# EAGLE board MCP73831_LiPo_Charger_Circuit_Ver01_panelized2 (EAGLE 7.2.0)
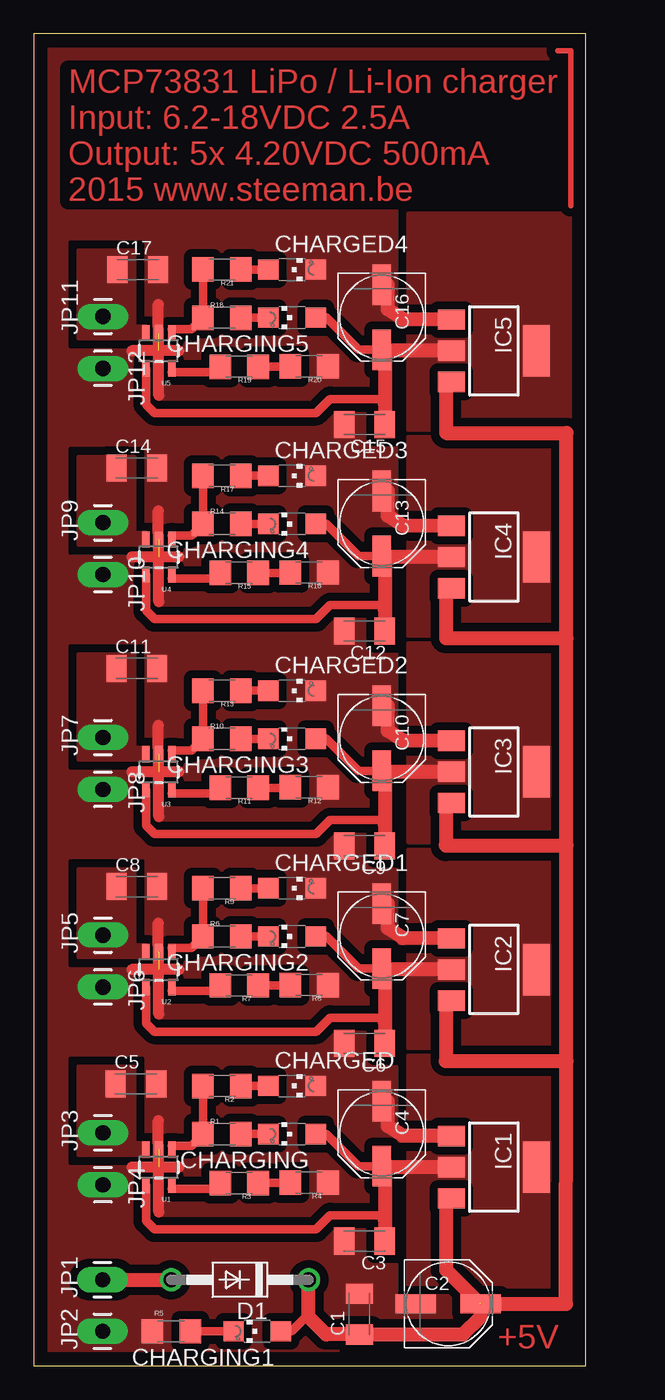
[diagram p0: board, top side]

Size 40.81 x 98.42 mm. Coordinates in mm from the lower left corner, seen from the top.
Outline: 0,0 40.81,0 40.81,98.42 0,98.42 0,0
Copper layers (1*16): Top 0.035mm / dielectric 1.5mm / Bottom 0.035mm
Design rules "default": minimum track width 10mil, minimum drill 24mil, track to track 8mil, track to pad 8mil, pad to pad 8mil, via to via 8mil, smd to smd 8mil, copper to edge 40mil, drill to drill 8mil, minimum pad ring 10mil, minimum via ring 8mil, stop-mask expansion 4mil, vias tented up to drill 0mil, thermal gap 10mil

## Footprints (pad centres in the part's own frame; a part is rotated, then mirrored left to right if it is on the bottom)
C1206K = smd 1.5 x 2: 1 -1.5,0; 2 1.5,0
PANASONIC_D = smd 3 x 1.4: + 2.4,0; - -2.4,0
CHIPLED_1206 = smd 1.5 x 1.5: A 0,-1.75; C 0,1.75
DO41-10 = drill 1.118: A 5.08,0; C -5.08,0
SOT223 = smd 1.5 x 2: 1 -2.3,-3.15; 2 0,-3.15; 3 2.3,-3.15 | smd 3.8 x 2: 4 0,3.15
1X01_LONGPAD = drill 1.118 pad 1.88 long: 1 0,0
1206 = smd 1.6 x 1.8: 1 -1.4,0; 2 1.4,0
SOT23-5 = smd 0.55 x 1.2: 1 -0.95,-1.3; 2 0,-1.3; 3 0.95,-1.3; 4 0.95,1.3; 5 -0.95,1.3

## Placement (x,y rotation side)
C1  100n  [C1206K]  24.07,3.81 90 top
C2  [PANASONIC_D]  30.64,4.57 0 top
C3  100n  [C1206K]  24.45,9.21 180 top
C4  [PANASONIC_D]  25.72,17.14 270 top
C5  10µ  [C1206K]  7.56,20.83 0 top
C6  100n  [C1206K]  24.45,23.81 180 top
C7  [PANASONIC_D]  25.72,31.75 270 top
C8  10µ  [C1206K]  7.62,35.4 0 top
C9  100n  [C1206K]  24.45,38.42 180 top
C10  [PANASONIC_D]  25.72,46.35 270 top
C11  10µ  [C1206K]  7.62,51.53 0 top
C12  100n  [C1206K]  24.45,54.29 180 top
C13  [PANASONIC_D]  25.72,62.23 270 top
C14  10µ  [C1206K]  7.62,66.33 0 top
C15  100n  [C1206K]  24.45,69.53 180 top
C16  [PANASONIC_D]  25.72,77.47 270 top
C17  10µ  [C1206K]  7.68,80.99 0 top
CHARGED  [CHIPLED_1206]  19.08,20.67 270 top
CHARGED1  [CHIPLED_1206]  19.08,35.27 270 top
CHARGED2  [CHIPLED_1206]  19.08,49.88 270 top
CHARGED3  [CHIPLED_1206]  19.08,65.75 270 top
CHARGED4  [CHIPLED_1206]  19.08,80.99 270 top
CHARGING  [CHIPLED_1206]  19.08,17.11 90 top
CHARGING1  [CHIPLED_1206]  16.51,2.54 90 top
CHARGING2  [CHIPLED_1206]  19.08,31.72 90 top
CHARGING3  [CHIPLED_1206]  19.08,46.32 90 top
CHARGING4  [CHIPLED_1206]  19.08,62.2 90 top
CHARGING5  [CHIPLED_1206]  19.08,77.44 90 top
D1  1N4004  [DO41-10]  15.24,6.35 180 top
IC1  TLV1117-50IDCYR (2342579)  [SOT223]  34,14.67 270 top
IC2  TLV1117-50IDCYR (2342579)  [SOT223]  34,29.27 270 top
IC3  TLV1117-50IDCYR (2342579)  [SOT223]  34,43.88 270 top
IC4  TLV1117-50IDCYR (2342579)  [SOT223]  34,59.75 270 top
IC5  TLV1117-50IDCYR (2342579)  [SOT223]  34,74.99 270 top
JP1  M01PTH_LONGPAD  [1X01_LONGPAD]  5.08,6.35 90 top
JP2  M01PTH_LONGPAD  [1X01_LONGPAD]  5.08,2.54 90 top
JP3  M01PTH_LONGPAD  [1X01_LONGPAD]  5.11,17.21 90 top
JP4  M01PTH_LONGPAD  [1X01_LONGPAD]  5.11,13.37 270 top
JP5  M01PTH_LONGPAD  [1X01_LONGPAD]  5.11,31.81 90 top
JP6  M01PTH_LONGPAD  [1X01_LONGPAD]  5.11,27.97 270 top
JP7  M01PTH_LONGPAD  [1X01_LONGPAD]  5.11,46.42 90 top
JP8  M01PTH_LONGPAD  [1X01_LONGPAD]  5.11,42.58 270 top
JP9  M01PTH_LONGPAD  [1X01_LONGPAD]  5.11,62.29 90 top
JP10  M01PTH_LONGPAD  [1X01_LONGPAD]  5.11,58.45 270 top
JP11  M01PTH_LONGPAD  [1X01_LONGPAD]  5.11,77.53 90 top
JP12  M01PTH_LONGPAD  [1X01_LONGPAD]  5.11,73.69 270 top
R1  1K  [1206]  13.91,17.11 0 top
R2  1K  [1206]  13.91,20.67 180 top
R3  1K  [1206]  15.18,13.49 180 top
R4  1K  [1206]  20.35,13.53 180 top
R5  1K  [1206]  10.16,2.54 0 top
R6  1K  [1206]  13.91,31.72 0 top
R7  1K  [1206]  15.18,28.1 180 top
R8  1K  [1206]  20.35,28.13 180 top
R9  1K  [1206]  13.91,35.27 180 top
R10  1K  [1206]  13.91,46.32 0 top
R11  1K  [1206]  15.18,42.7 180 top
R12  1K  [1206]  20.35,42.74 180 top
R13  1K  [1206]  13.91,49.88 180 top
R14  1K  [1206]  13.91,62.2 0 top
R15  1K  [1206]  15.18,58.58 180 top
R16  1K  [1206]  20.35,58.61 180 top
R17  1K  [1206]  13.91,65.75 180 top
R18  1K  [1206]  13.91,77.44 0 top
R19  1K  [1206]  15.18,73.82 180 top
R20  1K  [1206]  20.35,73.85 180 top
R21  1K  [1206]  13.91,80.99 180 top
U1  MCP73831  [SOT23-5]  9.24,14.67 180 top
U2  MCP73831  [SOT23-5]  9.24,29.27 180 top
U3  MCP73831  [SOT23-5]  9.24,43.88 180 top
U4  MCP73831  [SOT23-5]  9.24,59.75 180 top
U5  MCP73831  [SOT23-5]  9.24,74.99 180 top

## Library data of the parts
C1-C17 = rcl
CHARGED CHARGED1-CHARGED4 CHARGING CHARGING1-CHARGING5 = adafruit
D1 = diode
IC1-IC5 = v-reg
JP1-JP12 R1-R21 U1-U5 = SparkFun

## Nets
GND: C1.2 C2.- C3.2 C4.- C5.2 C6.2 C7.- C8.2 C9.2 C10.- C11.2 C12.2 C13.- C14.2 C15.2 C16.- C17.2 CHARGED1.C CHARGED2.C CHARGED3.C CHARGED4.C CHARGED.C IC1.1 IC2.1 IC3.1 IC4.1 IC5.1 JP2.1 JP4.1 JP6.1 JP8.1 JP10.1 JP12.1 R4.1 R5.1 R8.1 R12.1 R16.1 R20.1 U1.2 U2.2 U3.2 U4.2 U5.2
LIPO: C5.1 JP3.1 U1.3
LIPO1: C8.1 JP5.1 U2.3
LIPO2: C11.1 JP7.1 U3.3
LIPO3: C14.1 JP9.1 U4.3
LIPO5: C17.1 JP11.1 U5.3
N$1: CHARGING1.C R5.2
N$2: R3.1 R4.2
N$3: CHARGING.C R1.2
N$4: R3.2 U1.5
N$5: R1.1 R2.2 U1.1
N$6: CHARGED.A R2.1
N$7: CHARGING2.C R6.2
N$8: R7.1 R8.2
N$9: R7.2 U2.5
N$10: R6.1 R9.2 U2.1
N$11: CHARGED1.A R9.1
N$12: CHARGING3.C R10.2
N$13: R11.1 R12.2
N$14: R11.2 U3.5
N$15: R10.1 R13.2 U3.1
N$16: CHARGED2.A R13.1
N$17: CHARGING4.C R14.2
N$18: R15.1 R16.2
N$19: R15.2 U4.5
N$20: R14.1 R17.2 U4.1
N$21: CHARGED3.A R17.1
N$22: CHARGING5.C R18.2
N$23: R19.1 R20.2
N$24: R19.2 U5.5
N$25: R18.1 R21.2 U5.1
N$26: CHARGED4.A R21.1
V_IN: D1.A JP1.1
V_IN_PROT: C1.1 C2.+ CHARGING1.A D1.C IC1.3 IC4.3
V_IN_PROT1: IC2.3
V_IN_PROT2: IC3.3
V_IN_PROT4: IC5.3
VCC: C3.1 C4.+ CHARGING.A IC1.2 IC1.4 U1.4
VCC1: C6.1 C7.+ CHARGING2.A IC2.2 IC2.4 U2.4
VCC2: C9.1 C10.+ CHARGING3.A IC3.2 IC3.4 U3.4
VCC3: C12.1 C13.+ CHARGING4.A IC4.2 IC4.4 U4.4
VCC5: C15.1 C16.+ CHARGING5.A IC5.2 IC5.4 U5.4

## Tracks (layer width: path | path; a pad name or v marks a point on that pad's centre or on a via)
GND  (5 unrouted)
  Top 0.813: 9.24,11.37 9.24,14.67 9.21,18.1 | 10.73,14.67 7.24,14.67 | 9.24,25.97 9.24,29.27 9.21,32.7 | 10.73,29.27 7.24,29.27 | 9.24,40.58 9.24,43.88 9.21,47.31 | 10.73,43.88 7.24,43.88 | 9.24,56.45 9.24,59.75 9.21,63.18 | 10.73,59.75 7.24,59.75 | 9.24,71.69 9.24,74.99 9.21,78.42 | 10.73,74.99 7.24,74.99
  Top 1.016: IC1.1 27.28,17 26.16,17.72 26.16,19.55 C4.- | IC2.1 27.28,31.61 26.16,32.32 26.16,34.15 C7.- | IC3.1 27.28,46.21 26.16,46.93 26.16,48.76 C10.- | IC4.1 27.28,62.09 26.16,62.8 26.16,64.63 C13.- | IC5.1 27.28,77.33 26.16,78.04 26.16,79.87 C16.-
  pour Top (isolate 0.61, rank 2, no thermals): 0,0 0,99.06 40.64,99.06 40.64,0
LIPO
  pour Top (isolate 0.254, no thermals): 8.29,15.56 3.27,15.56 3.27,22.1 7.46,22.1 7.46,16.48 8.29,16.48
LIPO1
  pour Top (isolate 0.254, no thermals): 8.29,30.16 3.27,30.16 3.27,36.7 7.46,36.7 7.46,31.08 8.29,31.08
LIPO2
  pour Top (isolate 0.254, no thermals): 8.29,44.77 3.27,44.77 3.27,52.58 7.46,52.58 7.46,45.69 8.29,45.69
LIPO3
  pour Top (isolate 0.254, no thermals): 8.29,60.64 3.27,60.64 3.27,67.18 7.46,67.18 7.46,61.56 8.29,61.56
LIPO5
  pour Top (isolate 0.254, no thermals): 8.29,75.88 3.27,75.88 3.27,82.42 7.46,82.42 7.46,76.8 8.29,76.8
N$1
  Top 0.61: R5.2 CHARGING1.C
N$2
  Top 0.61: R3.1 18.95,13.49 R4.2
N$3
  Top 0.61: CHARGING.C R1.2
N$4
  Top 0.406: 10.2,13.08 U1.5
  Top 0.61: 10.2,13.08 13.78,13.08 R3.2
N$5
  Top 0.254: U1.1 10.19,16.26
  Top 0.61: R2.2 R1.1 11.65,16.26 10.19,16.26
N$6
  Top 0.61: CHARGED.A R2.1
N$7
  Top 0.61: CHARGING2.C R6.2
N$8
  Top 0.61: R7.1 18.95,28.1 R8.2
N$9
  Top 0.406: 10.2,27.69 U2.5
  Top 0.61: 10.2,27.69 13.78,27.69 R7.2
N$10
  Top 0.254: U2.1 10.19,30.86
  Top 0.61: R9.2 R6.1 11.65,30.86 10.19,30.86
N$11
  Top 0.61: CHARGED1.A R9.1
N$12
  Top 0.61: CHARGING3.C R10.2
N$13
  Top 0.61: R11.1 18.95,42.7 R12.2
N$14
  Top 0.406: 10.2,42.29 U3.5
  Top 0.61: 10.2,42.29 13.78,42.29 R11.2
N$15
  Top 0.254: U3.1 10.19,45.47
  Top 0.61: R13.2 R10.1 11.65,45.47 10.19,45.47
N$16
  Top 0.61: CHARGED2.A R13.1
N$17
  Top 0.61: CHARGING4.C R14.2
N$18
  Top 0.61: R15.1 18.95,58.58 R16.2
N$19
  Top 0.406: 10.2,58.17 U4.5
  Top 0.61: 10.2,58.17 13.78,58.17 R15.2
N$20
  Top 0.254: U4.1 10.19,61.34
  Top 0.61: R17.2 R14.1 11.65,61.34 10.19,61.34
N$21
  Top 0.61: CHARGED3.A R17.1
N$22
  Top 0.61: CHARGING5.C R18.2
N$23
  Top 0.406: 18.95,73.82 R20.2
  Top 0.61: R19.1 18.95,73.82
N$24
  Top 0.406: 10.2,73.41 U5.5
  Top 0.61: 10.2,73.41 13.78,73.41 R19.2
N$25
  Top 0.254: U5.1 10.19,76.58
  Top 0.61: R21.2 R18.1 11.65,76.58 10.19,76.58
N$26
  Top 0.61: CHARGED4.A R21.1
S$1
  Top 0.406: 38.73,97.16 39.69,97.16 39.69,85.72
V_IN
  Top 1.016: JP1.1 D1.A
V_IN_PROT  (1 unrouted)
  Top 0.406: 20.32,3.81 D1.C
  Top 0.61: CHARGING1.A 19.05,2.54 20.32,3.81
  Top 1.016: D1.C 20.32,3.6 21.61,2.31 C1.1 31.73,2.31 33.04,3.62 C2.+ | 39.37,22.51 39.34,4.57 32.99,4.57 30.48,7.08 30.48,12.37 IC1.3 | 39.37,22.51 39.37,38.45 | 39.37,38.45 39.37,53.75 | 39.37,53.75 39.37,68.93 30.48,68.93 | IC4.3 30.48,57.45 30.48,53.75 39.37,53.75 | 30.45,38.45 39.37,38.45 | 30.45,22.51 39.37,22.51
V_IN_PROT1
  Top 1.016: IC2.3 30.48,26.97 30.48,22.54
V_IN_PROT2
  Top 1.016: IC3.3 30.48,41.58 30.48,38.42
V_IN_PROT4
  Top 1.016: IC5.3 30.48,72.69 30.48,68.96
VCC
  Top 0.61: U1.4 8.29,10.7 8.91,10.07 20.87,10.07 21.91,11.11 25.95,11.11 25.95,10.79 | C4.+ 23.99,14.74 21.59,17.14 20.86,17.14 CHARGING.A
  Top 1.016: IC1.2 25.95,14.67 | C4.+ 25.79,14.67 25.95,14.67 | 25.95,14.67 25.95,10.79 C3.1
  pour Top (isolate 0.61, no thermals): 40.35,5.65 27.65,5.65 27.65,22.92 40.35,22.92
VCC1
  Top 0.61: U2.4 8.29,25.3 8.91,24.68 20.87,24.68 21.91,25.72 25.95,25.72 25.95,25.4 | C7.+ 23.99,29.35 21.59,31.75 20.86,31.75 CHARGING2.A
  Top 1.016: IC2.2 25.95,29.27 | C7.+ 25.79,29.27 25.95,29.27 | 25.95,29.27 25.95,25.4 C6.1
  pour Top (isolate 0.61, no thermals): 40.35,23.43 27.65,23.43 27.65,38.16 40.35,38.16
VCC2
  Top 0.61: U3.4 8.29,39.91 8.91,39.28 20.87,39.28 21.91,40.32 25.95,40.32 25.95,40.01 | C10.+ 23.99,43.95 21.59,46.35 20.86,46.35 CHARGING3.A
  Top 1.016: IC3.2 25.95,43.88 | C10.+ 25.79,43.88 25.95,43.88 | 25.95,43.88 25.95,40.01 C9.1
  pour Top (isolate 0.61, no thermals): 40.35,38.67 27.65,38.67 27.65,53.4 40.35,53.4
VCC3
  Top 0.61: U4.4 8.29,55.78 8.91,55.16 20.87,55.16 21.91,56.2 25.95,56.2 25.95,55.88 | C13.+ 23.99,59.83 21.59,62.23 20.86,62.23 CHARGING4.A
  Top 1.016: IC4.2 25.95,59.75 | C13.+ 25.79,59.75 25.95,59.75 | 25.95,59.75 25.95,55.88 C12.1
  pour Top (isolate 0.61, no thermals): 40.35,53.91 27.65,53.91 27.65,68.64 40.35,68.64
VCC5
  Top 0.61: U5.4 8.29,71.03 8.91,70.4 20.87,70.4 21.91,71.44 25.95,71.44 25.95,71.12 | C16.+ 23.99,75.07 21.59,77.47 20.86,77.47 CHARGING5.A
  Top 1.016: IC5.2 25.95,74.99 | C16.+ 25.79,74.99 25.95,74.99 | 25.95,74.99 25.95,71.12 C15.1
  pour Top (isolate 0.61, no thermals): 40.35,69.15 27.65,69.15 27.65,85.15 40.35,85.15

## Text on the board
Top: MCP73831 LiPo / Li-Ion charger / Input: 6.2-18VDC 2.5A / Output: 5x 4.20VDC 500mA / 2015 www.steeman.be | +5V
